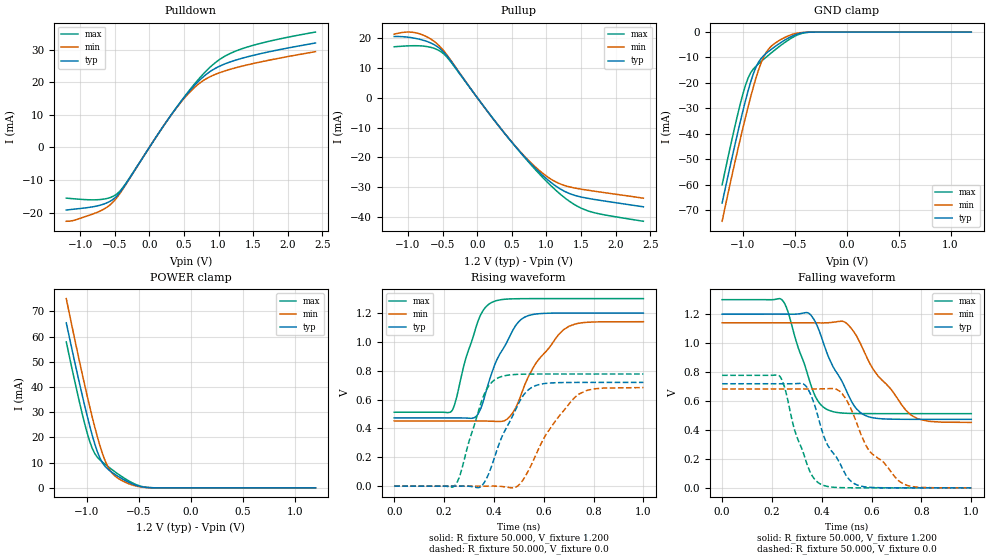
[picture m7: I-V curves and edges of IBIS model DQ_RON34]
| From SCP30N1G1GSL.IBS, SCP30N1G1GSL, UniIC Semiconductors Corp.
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|   Model DQ_RON34
[Model] DQ_RON34
Model_type I/O
Vinl =  0.500V
Vinh =  0.700V
Vmeas =  0.600V
Rref =  50.000
Vref =  0.600V
C_comp   1.373pF   1.353pF   1.403pF
[Model Spec]
Vinh   0.700V   0.670V   0.750V
Vinl   0.500V   0.470V   0.550V
Vmeas   0.600V   0.570V   0.650V
Vref   0.600V   0.570V   0.650V
Rref   50.000   NA   NA
[Temperature Range]   25.000   85.000   -40.000
[Voltage Range]   1.200V   1.140V   1.300V
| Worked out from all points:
|   slope of the pulldown table from 0 to 0.18 V, typ, clamps not added: 30.8 ohm
|   slope of the pullup table from 0 to 0.18 V, typ, clamps not added: 32.3 ohm
|   GND clamp passes 1 mA (typ) near -0.49 V on its own axis
|   POWER clamp passes 1 mA (typ) near -0.53 V on its own axis
|   rising waveform, R_fixture 50.000, V_fixture 1.200: 20-80 % time 106ps typ, 140ps min, 78.3ps max; typ from 0.473 V to 1.2 V
|   rising waveform, R_fixture 50.000, V_fixture 0.0: 20-80 % time 108ps typ, 144ps min, 80.9ps max; typ from 0 V to 0.719 V
|   falling waveform, R_fixture 50.000, V_fixture 1.200: 20-80 % time 117ps typ, 161ps min, 88.2ps max; typ from 1.2 V to 0.473 V
|   falling waveform, R_fixture 50.000, V_fixture 0.0: 20-80 % time 109ps typ, 150ps min, 81ps max; typ from 0.719 V to 0 V
[Pulldown]
|Voltage   I(typ)   I(min)   I(max)
-1.2V     -19.25mA   -22.7mA    -15.59mA
-719mV    -17.8mA    -19.62mA   -16.03mA
-571mV    -16.59mA   -17.71mA   -15.44mA
-460mV    -14.71mA   -15.18mA   -14.13mA
-349mV    -11.55mA   -11.7mA    -11.33mA
317mV     10.05mA    10mA       10.04mA
576mV     17.23mA    16.81mA    17.49mA
761mV     21.36mA    20.29mA    22.15mA
1.02V     25.02mA    23mA       27.1mA
1.279V    27.04mA    24.66mA    29.87mA
1.723V    29.37mA    26.79mA    32.59mA
2.4V      32.1mA     29.44mA    35.47mA
[Pullup]
|Voltage   I(typ)   I(min)   I(max)
-1.2V     20.45mA    21.24mA    17.03mA
-1.004V   20.23mA    21.95mA    17.32mA
-819mV    19.45mA    21.25mA    17.32mA
-634mV    17.86mA    19.02mA    16.59mA
-486mV    15.25mA    15.73mA    14.68mA
69mV      -2.161mA   -2.176mA   -2.131mA
439mV     -13.2mA    -13.18mA   -13.17mA
772mV     -22.04mA   -21.69mA   -22.33mA
1.031V    -27.73mA   -26.74mA   -28.69mA
1.29V     -31.65mA   -29.58mA   -33.96mA
1.549V    -33.46mA   -30.79mA   -37.44mA
2.4V      -36.51mA   -33.63mA   -41.35mA
[GND_clamp]
|Voltage   I(typ)   I(min)   I(max)
-1.2V     -67.26mA   -74.42mA   -60.1mA
-1.05V    -39.62mA   -46.47mA   -32.4mA
-1V       -31.05mA   -37.77mA   -24.37mA
-950mV    -23.16mA   -29.46mA   -18.1mA
-925mV    -19.62mA   -25.5mA    -16.02mA
-875mV    -13.89mA   -18.21mA   -13.48mA
-825mV    -10.4mA    -12.16mA   -11.61mA
-775mV    -8.365mA   -7.964mA   -9.852mA
-700mV    -6.001mA   -4.671mA   -7.319mA
-525mV    -1.587mA   -933.3uA   -2.208mA
-375mV    -90.13uA   -49.22uA   -132.9uA
1.2V      0A         0A         0A
[POWER_clamp]
|Voltage   I(typ)   I(min)   I(max)
-1.2V     65.51mA    75.11mA    57.91mA
-1.05V    37.38mA    45.87mA    29.99mA
-1V       28.74mA    36.73mA    21.95mA
-950mV    20.85mA    28.08mA    15.65mA
-925mV    17.34mA    24.01mA    13.56mA
-875mV    11.74mA    16.61mA    11.06mA
-825mV    8.457mA    10.65mA    9.317mA
-775mV    6.603mA    6.7mA      7.708mA
-725mV    5.177mA    4.492mA    6.178mA
-550mV    1.336mA    943.1uA    1.707mA
-400mV    85.95uA    67.55uA    91.19uA
1.2V      0A         0A         0A
[Ramp]
| variable   typ   min   max
dV/dt_r   0.431/0.108n   0.410/0.144n   0.466/80.781p
dV/dt_f   0.436/0.117n   0.413/0.161n   0.472/87.928p
R_load = 50.000
[Rising Waveform]
R_fixture= 50.000
V_fixture= 1.200
V_fixture_min= 1.140
V_fixture_max= 1.300
|time   V(typ)   V(min)   V(max)
0s        473.3mV    451.9mV    512.6mV
232ps     473.4mV    451.9mV    523.2mV
331ps     487.7mV    452mV      1.117V
393ps     791.3mV    450mV      1.275V
453ps     1V         464.4mV    1.297V
507ps     1.152V     623mV      1.299V
566ps     1.193V     844.8mV    1.3V
679ps     1.2V       1.083V     1.3V
767ps     1.2V       1.135V     1.3V
1ns       1.2V       1.14V      1.3V
[Rising Waveform]
R_fixture= 50.000
V_fixture= 0.0
V_fixture_min= 0.0
V_fixture_max= 0.0
|time   V(typ)   V(min)   V(max)
0s        35.08nV    111.6nV    20.74nV
244ps     132.3uV    -11.82uV   5.093mV
265ps     422.7uV    -24.87uV   81.16mV
353ps     4.683mV    274.5uV    600.6mV
417ps     274.1mV    -46.59uV   750.9mV
494ps     554.7mV    -1.018mV   774.9mV
566ps     695.9mV    206.9mV    777.1mV
648ps     717mV      454.6mV    777.4mV
743ps     719mV      639.9mV    777.4mV
1ns       719.2mV    683.3mV    777.4mV
[Falling Waveform]
R_fixture= 50.000
V_fixture= 1.200
V_fixture_min= 1.140
V_fixture_max= 1.300
|time   V(typ)   V(min)   V(max)
0s        1.2V       1.14V      1.3V
240ps     1.2V       1.14V      1.3V
263ps     1.2V       1.14V      1.223V
357ps     1.193V     1.14V      706.1mV
427ps     903.8mV    1.141V     536.6mV
496ps     681.4mV    1.141V     515.3mV
568ps     505mV      948.8mV    512.9mV
627ps     478.8mV    770.2mV    512.7mV
757ps     473.4mV    503.8mV    512.6mV
1ns       473.3mV    452mV      512.6mV
[Falling Waveform]
R_fixture= 50.000
V_fixture= 0.0
V_fixture_min= 0.0
V_fixture_max= 0.0
|time   V(typ)   V(min)   V(max)
0s        719.2mV    683.3mV    777.4mV
233ps     719mV      683.3mV    768.2mV
292ps     719.7mV    683.3mV    392.9mV
337ps     702.3mV    683.1mV    182.8mV
398ps     411.3mV    683.7mV    23.23mV
477ps     154.3mV    659.4mV    1.381mV
543ps     18.8mV     434.4mV    128.1uV
593ps     3.311mV    251mV      21.1uV
726ps     32.33uV    28.32mV    187.1nV
1ns       33.66nV    5.18uV     17.71nV
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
